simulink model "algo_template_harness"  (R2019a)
settings: configuration reference "configurationSettings" (kept in a data dictionary, not in this file)
undefined symbols (not defined in the file or in its folder): algo_template_fp

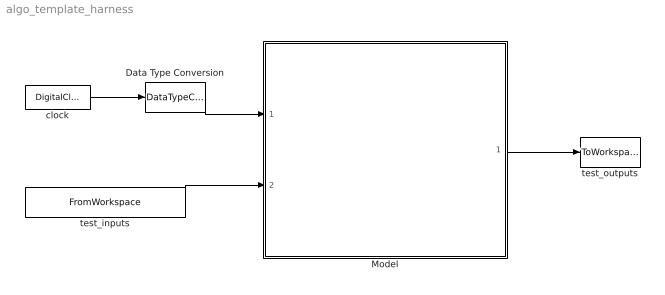
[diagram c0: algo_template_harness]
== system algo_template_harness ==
  Data Type Conversion : DataTypeConversion  OutDataTypeStr=single
  Model : ModelReference  ModelNameDialog=algo_template.slx  SimulationMode=Normal  ModelReferenceVersion=1.782  SimulationMode=Normal
  clock : DigitalClock  SampleTime=algo_template_fp.timing.dt
  test_inputs : FromWorkspace  VariableName=algo_template_inbus1  OutDataTypeStr=Bus: algo_template_inBus  SampleTime=algo_template_fp.timing.dt  Interpolate=off  OutputAfterFinalValue=Holding final value
  test_outputs : ToWorkspace  VariableName=simout  SaveFormat=Timeseries  SampleTime=-1
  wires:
  Model/1 -> test_outputs/1
  clock/1 -> Data Type Conversion/1
  test_inputs/1 -> Model/2
  Data Type Conversion/1 -> Model/1
